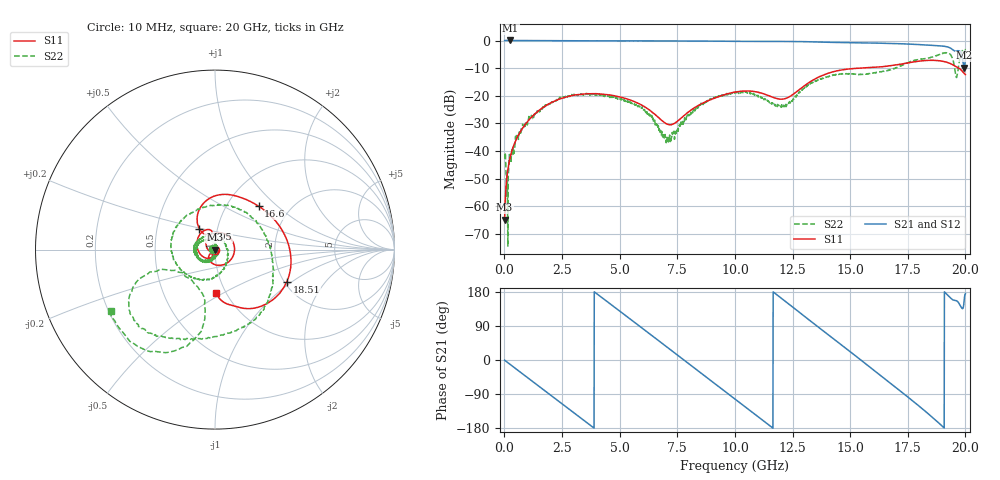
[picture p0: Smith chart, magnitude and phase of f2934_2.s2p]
!Keysight Technologies,M9372A,MY54321350,A.13.90.07
!Automatic Fixture Removal (AFR)
!Date: Wednesday, January 06, 2021, 09:20:31
!S2P File: Measurements: S11,S21,S12,S22:
# MHz S  RI  R 50
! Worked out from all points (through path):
!   2000 points, 10 MHz to 20 GHz, reference 50 ohm
!   highest |S21| = 0.03 dB at 260 MHz (marker M1); lowest = -9.8 dB at 19.94 GHz (marker M2)
!   group delay of S21, straight-line fit = 130 ps
!   lowest |S11| = -64.9 dB at 10 MHz (marker M3), VSWR 1.00, Z = 50 - j0.0296 ohm
!   |S11| at or under -10 dB: start of sweep to 15.41 GHz; 19.71 GHz to end of sweep
!   |S22| runs from -74.5 to -3.1 dB; largest |S21 - S12| = 1e-14
!   S11 on the Smith chart (normalised r, x): 10 MHz: 1.00, -0.00; 12.95 GHz: 0.82, +0.19; 16.6 GHz: 1.40, +0.77; 18.51 GHz: 2.06, -0.91; 20 GHz: 0.90, -0.46
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10  0.000485 -0.000296  1.001 -0.00797  1.001 -0.00797  -0.00863 0.000698
160  -0.000462 -0.00484  0.9944 -0.1293  0.9944 -0.1293  0.000297 0.000431
260  -0.00227 -0.00765  0.9814 -0.2101  0.9814 -0.2101  -0.000112 -0.00708
740  -0.0207 -0.0121  0.8273 -0.5649  0.8273 -0.5649  0.00163 -0.0231
1840  -0.046 0.0498  0.0819 -0.9941  0.0819 -0.9941  -0.0354 -0.0576
3350  0.0843 0.0655  -0.8956 -0.4209  -0.8956 -0.4209  -0.1043 -0.0232
5280  0.0143 -0.0873  -0.4372 0.8841  -0.4372 0.8841  -0.0593 0.053
6680  -0.0303 -0.027  0.6135 0.7716  0.6135 0.7716  0.00615 0.0277
7140  -0.018 -0.0239  0.8523 0.4945  0.8523 0.4945  0.0164 -0.000346
8180  -0.0317 -0.0488  0.931 -0.3072  0.931 -0.3072  -0.00571 -0.0524
10010  -0.0922 0.0711  -0.2217 -0.9423  -0.2217 -0.9423  -0.1112 -0.022
11530  -0.0155 0.0969  -0.959 -0.0995  -0.959 -0.0995  -0.0073 0.0765
12950  -0.0869 0.116  -0.456 0.8374  -0.456 0.8374  0.0295 -0.129
13340  -0.0996 0.1583  -0.1643 0.9329  -0.1643 0.9329  -0.0415 -0.1674
15110  0.0415 0.3073  0.8722 0.2632  0.8722 0.2632  -0.1818 0.168
16600  0.2431 0.2419  0.5224 -0.7211  0.5224 -0.7211  0.2633 0.1113
16670  0.2541 0.2346  0.4775 -0.7484  0.4775 -0.7484  0.2768 0.0856
18510  0.3999 -0.1795  -0.6959 -0.4343  -0.6959 -0.4343  -0.0555 -0.4949
19300  0.2137 -0.3271  -0.7288 0.1702  -0.7288 0.1702  -0.4789 -0.3348
19610  0.1111 -0.3149  -0.591 0.2568  -0.591 0.2568  -0.1476 -0.1585
19940  0.0135 -0.2552  -0.2881 0.1444  -0.2881 0.1444  -0.4945 -0.4844
20000  0.00719 -0.2409  -0.4424 0.0399  -0.4424 0.0399  -0.5806 -0.3441
